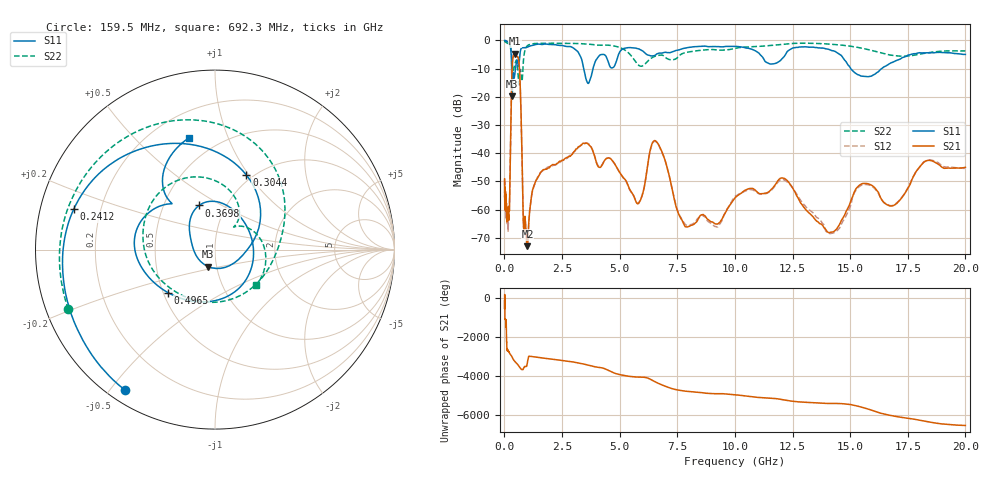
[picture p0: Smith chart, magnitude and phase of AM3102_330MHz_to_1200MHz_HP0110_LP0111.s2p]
! Date/Time: Tue, Sep 11, 2018 5:15 PM
! Network Analyzer: Agilent Technologies E8362B Rev: A.07.50.63
! Sweep from 0.010 to 20.000 GHz, 1601 Points, Sweep Type: LOG
! Power Supply: 4.949 V, 0.001 A
# Hz S DB R 50
!freq MagS11 AngS11 MagS21 AngS21 MagS12 AngS12 MagS22 AngS22
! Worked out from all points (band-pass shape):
!   1601 points, 10 MHz to 20 GHz, reference 50 ohm
!   highest |S21| = -4.74 dB at 445.1 MHz (marker M1); lowest = -72.9 dB at 1.003 GHz (marker M2)
!   |S21| within 3 dB of the highest: 349.1 MHz to 632.4 MHz (283.2 MHz wide, 57.7 % of centre)
!   lowest |S11| = -19.8 dB at 337.9 MHz (marker M3), VSWR 1.23, Z = 45.4 - j8.65 ohm
!   |S11| at or under -10 dB: 314.7 MHz to 483.1 MHz (168.3 MHz wide, 42.2 % of centre); 3.441 GHz to 3.842 GHz (401.5 MHz wide, 11 % of centre); 15.03 GHz to 16.37 GHz (1.341 GHz wide, 8.55 % of centre)
!   |S22| runs from -15.8 to -0.2 dB; largest |S21 - S12| = 0.01
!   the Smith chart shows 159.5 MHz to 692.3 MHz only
!   S11 on the Smith chart (normalised r, x): 159.5 MHz: 0.05, -0.55; 241.2 MHz: 0.10, +0.14; 304.4 MHz: 0.93, +0.97; 369.8 MHz: 0.75, +0.39; 496.5 MHz: 0.53, -0.29; 692.3 MHz: 0.35, +0.73
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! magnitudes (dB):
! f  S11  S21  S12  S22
! 10 MHz  0.0  -49.1  -51.7  -0.2
! 35.55 MHz  0.0  -58.4  -58.4  -0.4
! 126.4 MHz  -0.4  -63.1  -62.7  -0.9
! 159.5 MHz  -0.6  -60.6  -65.8  -1.1
! 241.2 MHz  -1.7  -49.9  -49.7  -1.7
! 304.4 MHz  -6.9  -19.4  -19.5  -3.9
! 337.9 MHz  -19.8  -9.3  -9.3  -8.0
! 369.8 MHz  -11.7  -6.2  -6.3  -10.6
! 445.1 MHz  -12.4  -4.7  -4.8  -8.7
! 447.2 MHz  -12.3  -4.7  -4.8  -8.6
! 496.5 MHz  -9.0  -5.0  -5.1  -7.4
! 692.3 MHz  -3.9  -17.4  -17.4  -10.3
! 833.3 MHz  -2.6  -66.3  -66.1  -6.6
! 1.003 GHz  -2.4  -72.9  -71.8  -1.9
! 1.59 GHz  -1.4  -46.6  -46.7  -1.0
! 3.582 GHz  -14.6  -36.5  -36.4  -1.3
! 5.652 GHz  -2.7  -55.9  -56.0  -7.1
! 6.58 GHz  -5.0  -35.7  -35.9  -5.5
! 7.92 GHz  -2.6  -66.1  -65.5  -4.2
! 12.03 GHz  -6.6  -48.7  -49.3  -1.4
! 14.21 GHz  -3.6  -67.9  -68.3  -1.4
! 20 GHz  -4.9  -45.0  -45.4  -3.7
